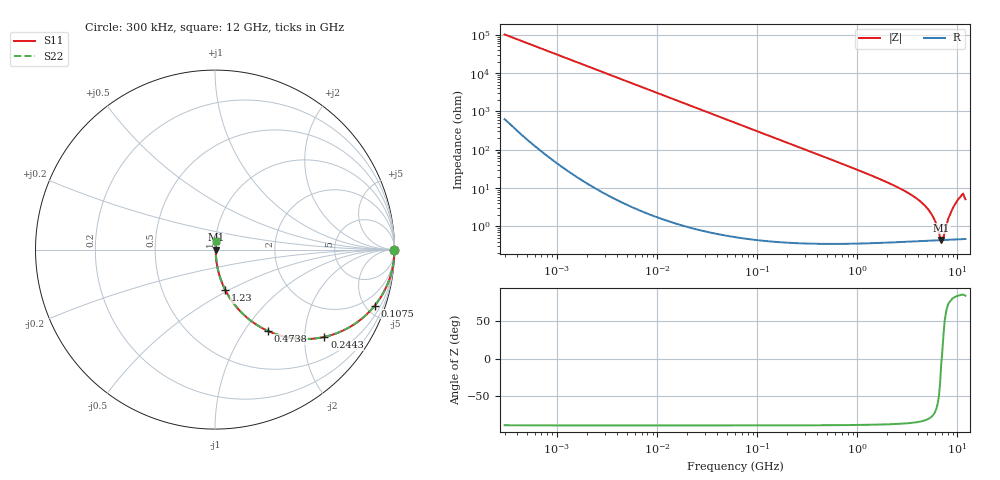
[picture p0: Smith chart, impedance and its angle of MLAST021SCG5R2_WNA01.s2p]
! MLAST021SCG5R2_WNA01  S-PARAMETER MODEL  ( General Type )
! Model Generated by TAIYO YUDEN Corporation (http://www.ty-top.com)
! Version 1.0
! TAIYO YUDEN Control No. 220901
! Copyright(c) 2022 TAIYO YUDEN CO.,LTD. All Rights Reserved.
! Product Description (link to TY-COMPAS)
! https://ds.yuden.co.jp/TYCOMPAS/or/detail?pn=MLAST021SCG5R2CWNA01&u=M
! Products Name : Multilayer Ceramic Capacitors
! Characteristics :
!  Capacitance : 5.2 pF , Rated Voltage : 25V , TCC : CG / C0G
!  Case Size : 0.25 x 0.125 / 0.0098 x 0.0049 [mm/inch] , Thickness : 0.125 / 0.0049 [mm/inch]
!  (Conditions: Temperature = 25 degC , DC Bias Current/Voltage = 0A / 0V)
! External Node Assignments :
!  1  o---| |---o  2
! GND o---------o GND
! Frequency Range : 0.3MHz  -  12000MHz  [ 401 STEP ]
# MHz S RI R 50
! Freq[MHz].  S11 Real  S11 Imag  S21 Real  S21 Imag  S12 Real  S12 Imag  S22 Real  S22 Imag
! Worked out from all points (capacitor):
!   401 points, 300 kHz to 12 GHz, reference 50 ohm
!   read as one part in series: C = 5.2 pF near 316.3 kHz
!   lowest |Z| = 444 mohm at 6.88 GHz (marker M1)
!   series resonance near 6.961 GHz, so ESL is about 100 pH
!   S11 on the Smith chart (normalised r, x): 300 kHz: open; 107.5 MHz: 1.01, -5.69; 244.3 MHz: 1.01, -2.50; 473.8 MHz: 1.01, -1.29; 1.23 GHz: 1.01, -0.48; 12 GHz: 1.01, +0.10
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0.3  1 -0.00098  6.98e-06 0.00098  6.98e-06 0.00098  1 -0.00098
1.769972  1 -0.00578  3.88e-05 0.00578  3.88e-05 0.00578  1 -0.00578
10.44266  0.9988 -0.0341  0.00118 0.0341  0.00118 0.0341  0.9988 -0.0341
27.82928  0.9917 -0.0902  0.00826 0.0902  0.00826 0.0902  0.9917 -0.0902
60  0.9628 -0.1887  0.0372 0.1887  0.0372 0.1887  0.9628 -0.1887
107.4644  0.8898 -0.3123  0.1102 0.3123  0.1102 0.3123  0.8898 -0.3123
159.8975  0.7849 -0.4098  0.2151 0.4098  0.2151 0.4098  0.7849 -0.4098
244.3004  0.6099 -0.4863  0.3901 0.4863  0.3901 0.4863  0.6099 -0.4863
353.9943  0.4268 -0.4926  0.5732 0.4926  0.5732 0.4926  0.4268 -0.4926
473.7541  0.2936 -0.4527  0.7064 0.4527  0.7064 0.4527  0.2936 -0.4527
743.2595  0.1443 -0.3471  0.8557 0.3471  0.8557 0.3471  0.1443 -0.3471
1229.528  0.058 -0.2263  0.942 0.2263  0.942 0.2263  0.058 -0.2263
2088.533  0.021 -0.1299  0.979 0.1299  0.979 0.1299  0.021 -0.1299
3454.93  0.00837 -0.0657  0.9916 0.0657  0.9916 0.0657  0.00837 -0.0657
4747.894  0.00533 -0.0339  0.9947 0.0339  0.9947 0.0339  0.00533 -0.0339
5715.274  0.00457 -0.017  0.9954 0.017  0.9954 0.017  0.00457 -0.017
6879.757  0.00438 -0.000609  0.9956 0.000609  0.9956 0.000609  0.00438 -0.000609
7254.098  0.00441 0.00277  0.9956 -0.00277  0.9956 -0.00277  0.00441 0.00277
8281.503  0.00478 0.0174  0.9952 -0.0174  0.9952 -0.0174  0.00478 0.0174
9454.42  0.00593 0.0371  0.9941 -0.0371  0.9941 -0.0371  0.00593 0.0371
10793.46  0.00818 0.0595  0.9918 -0.0595  0.9918 -0.0595  0.00818 0.0595
12000  0.00721 0.0502  0.9928 -0.0502  0.9928 -0.0502  0.00721 0.0502
